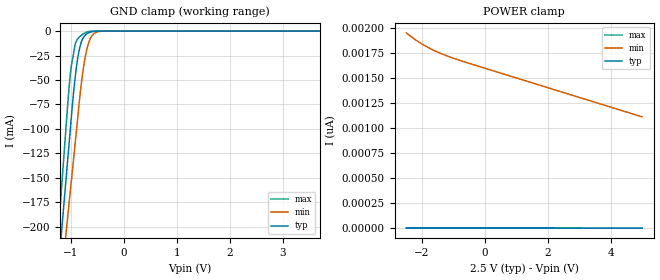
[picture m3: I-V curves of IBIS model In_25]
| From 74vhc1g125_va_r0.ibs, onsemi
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|//////////////////////////////////////////////////////////////////////////////
|//////////////////////////////////////////////////////////////////////////////
[Model]  In_25
Model_type Input
Vinh =  1.75
Vinl =  0.75
|  variable   typ   min   max
C_comp   2.7pF   2.7pF   2.7pF
|//////////////////////////////////////////////////////////////////////////////
[Temperature Range]   25   125   -55
|//////////////////////////////////////////////////////////////////////////////
[Voltage Range]   2.50V   2.30V   2.70V
|//////////////////////////////////////////////////////////////////////////////
[POWER Clamp Reference] 2.50V   2.30V   2.70V
|//////////////////////////////////////////////////////////////////////////////
[GND Clamp Reference]   0V   0V   0V
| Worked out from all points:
|   GND clamp passes 1 mA (typ) near -0.63 V on its own axis
|//////////////////////////////////////////////////////////////////////////////
[GND Clamp]
|   Voltage   I(typ)   I(min)   I(max)
-2.5V     -1.041A    -954mA     -1.13A
-1.28V    -269.1mA   -305.4mA   -234.4mA
-1.22V    -231.1mA   -273.5mA   -190.4mA
-1.16V    -193.2mA   -241.6mA   -146.3mA
-1.08V    -142.6mA   -199.1mA   -87.64mA
-1V       -91.95mA   -156.6mA   -37.57mA
-880mV    -29.98mA   -92.77mA   -8.501mA
-820mV    -13.68mA   -60.4mA    -4.947mA
-740mV    -4.627mA   -28.93mA   -1.931mA
-620mV    -868.6uA   -6.083mA   -115.8uA
-440mV    -5.78uA    -234.3uA   -25.3nA
5V        1.379pA    1.86nA     509.7fA
|//////////////////////////////////////////////////////////////////////////////
[POWER Clamp]
|   Voltage   I(typ)   I(min)   I(max)
-2.5V     1.379pA    1.952nA    517.7fA
-2.2V     1.326pA    1.88nA     501.8fA
-1.8V     1.255pA    1.805nA    469.9fA
-1.4V     1.184pA    1.746nA    438.1fA
-1V       1.113pA    1.698nA    406.3fA
5V        49.27fA    1.113nA    -71.19fA
